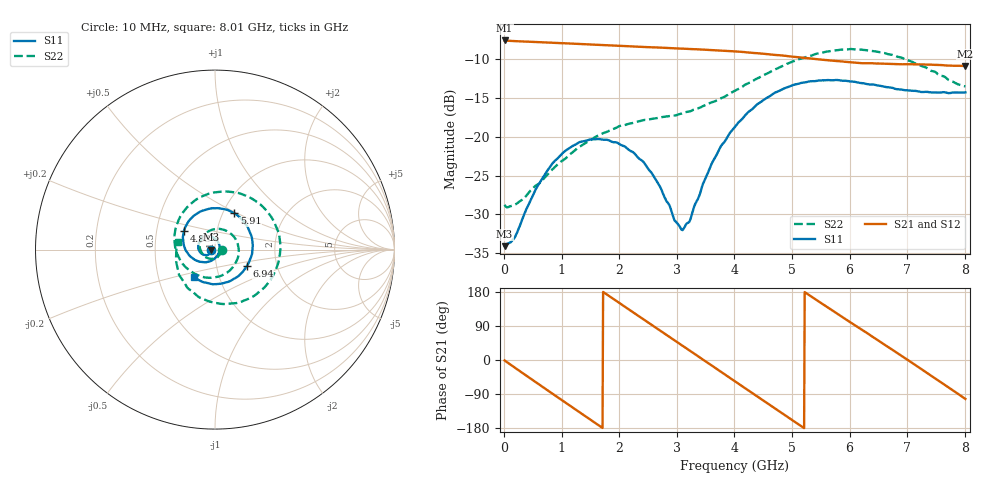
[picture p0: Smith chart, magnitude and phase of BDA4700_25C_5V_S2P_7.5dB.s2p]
!Agilent Technologies,E5071B,MY42404982,A.09.10
!Date: Mon Oct 20 13:29:44 2025
!Data & Calibration Information:
!Freq	S11:SOLT2(ON)	S21:SOLT2(ON)	S12:SOLT2(ON)	S22:SOLT2(ON)
# Hz S RI R 50
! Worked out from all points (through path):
!   801 points, 10 MHz to 8.01 GHz, reference 50 ohm
!   highest |S21| = -7.61 dB at 10 MHz (marker M1); lowest = -10.9 dB at 8.01 GHz (marker M2)
!   group delay of S21, straight-line fit = 285 ps
!   lowest |S11| = -34.1 dB at 10 MHz (marker M3), VSWR 1.04, Z = 48.1 - j0.0867 ohm
!   |S11| at or under -10 dB: start of sweep to end of sweep
!   |S22| runs from -29.1 to -8.7 dB; largest |S21 - S12| = 0.0032
!   S11 on the Smith chart (normalised r, x): 10 MHz: 0.96, -0.00; 4.83 GHz: 0.69, +0.15; 5.91 GHz: 1.13, +0.48; 6.94 GHz: 1.40, -0.27; 8.01 GHz: 0.76, -0.24
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1e7  -0.0198 -0.000901  0.4161 -0.00879  0.4162 -0.00939  0.0364 -0.00278
3.3e8  -0.0245 -0.0179  0.3348 -0.2366  0.3346 -0.2369  0.0238 -0.0317
7.2e8  -0.049 -0.0311  0.0961 -0.3924  0.096 -0.3925  -0.0197 -0.0517
1.02e9  -0.0754 -0.0223  -0.1206 -0.3807  -0.1205 -0.3811  -0.0618 -0.0338
1.35e9  -0.093 0.00614  -0.3104 -0.2432  -0.3106 -0.2437  -0.0852 0.0223
1.64e9  -0.0889 0.0383  -0.3861 -0.054  -0.3863 -0.0541  -0.0643 0.0791
1.93e9  -0.0665 0.0638  -0.3572 0.1447  -0.3571 0.1449  -0.00528 0.1133
2.32e9  -0.0224 0.0703  -0.1765 0.3358  -0.1764 0.3359  0.0885 0.0885
2.68e9  0.0139 0.0478  0.0605 0.3699  0.0607 0.3695  0.1322 1.37e-05
3.11e9  0.0245 -0.0068  0.2965 0.2186  0.2959 0.2192  0.0845 -0.1142
3.54e9  -0.0123 -0.0572  0.3588 -0.0491  0.3587 -0.0497  -0.0436 -0.1564
4.01e9  -0.0967 -0.0636  0.1963 -0.2943  0.1962 -0.294  -0.1827 -0.0757
4.41e9  -0.163 -0.00469  -0.0464 -0.341  -0.0462 -0.3419  -0.2264 0.0753
4.83e9  -0.1725 0.1049  -0.2587 -0.2098  -0.2578 -0.2105  -0.1489 0.2426
5.35e9  -0.0706 0.2165  -0.3084 0.077  -0.3088 0.0762  0.0948 0.3204
5.91e9  0.1072 0.2026  -0.1018 0.2861  -0.1024 0.286  0.3337 0.1442
6.28e9  0.187 0.1143  0.0848 0.2844  0.0873 0.2831  0.3553 -0.0624
6.68e9  0.2074 -0.0161  0.2463 0.1606  0.247 0.1601  0.2363 -0.244
6.94e9  0.1769 -0.093  0.2901 0.0367  0.2904 0.0353  0.1078 -0.2987
7.29e9  0.0941 -0.1697  0.2562 -0.1393  0.256 -0.14  -0.0759 -0.2716
7.6e9  -0.000623 -0.1929  0.1424 -0.2516  0.1419 -0.2518  -0.1905 -0.1559
8.01e9  -0.1187 -0.1521  -0.0631 -0.2778  -0.0631 -0.278  -0.2063 0.0437
